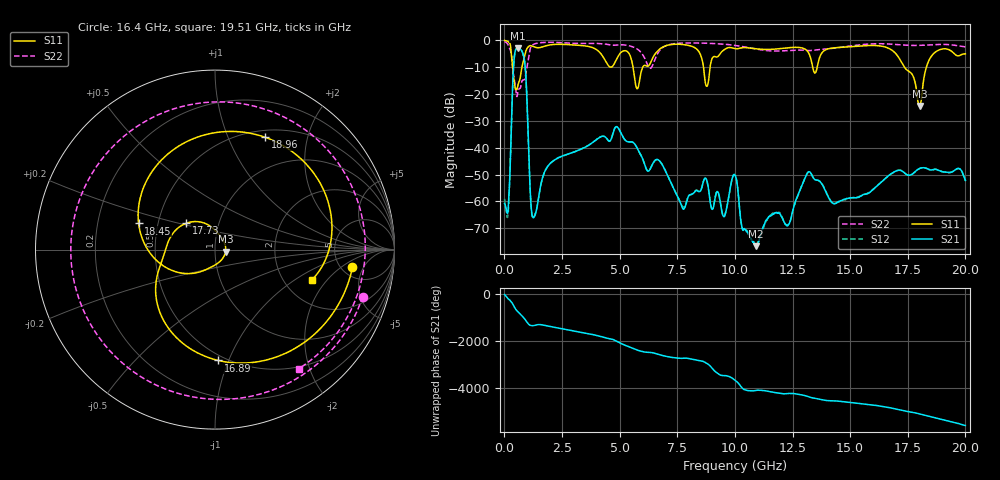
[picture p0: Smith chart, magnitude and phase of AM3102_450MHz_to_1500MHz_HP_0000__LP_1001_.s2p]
!Agilent Technologies,E8364B,MY43040894,A.07.50.67
!Agilent E8364B: A.07.50.67
!Date: Thursday, January 11, 2018 05:16:58
!Correction: S11(Full 2 Port(1,2))
!S21(Full 2 Port(1,2))
!S12(Full 2 Port(1,2))
!S22(Full 2 Port(1,2))
!S2P File: Measurements: S11, S21, S12, S22:
# Hz S  dB  R 50
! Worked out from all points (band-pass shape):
!   1601 points, 10 MHz to 20 GHz, reference 50 ohm
!   highest |S21| = -2.93 dB at 584.7 MHz (marker M1); lowest = -76.7 dB at 10.93 GHz (marker M2)
!   |S21| within 3 dB of the highest: 434.5 MHz to 835.3 MHz (400.8 MHz wide, 63.1 % of centre)
!   lowest |S11| = -24.5 dB at 18.01 GHz (marker M3), VSWR 1.13, Z = 56.2 - j1.29 ohm
!   |S11| at or under -10 dB: 355.9 MHz to 762.5 MHz (406.5 MHz wide, 72.7 % of centre); 5.581 GHz to 6.002 GHz (421.3 MHz wide, 7.28 % of centre); 17.35 GHz to 18.31 GHz (953 MHz wide, 5.34 % of centre)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
!   |S22| runs from -21.0 to -0.5 dB; largest |S21 - S12| = 0.0015
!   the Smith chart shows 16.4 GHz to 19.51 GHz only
!   S11 on the Smith chart (normalised r, x): 16.4 GHz: 6.27, -3.05; 16.89 GHz: 0.46, -0.92; 17.73 GHz: 0.70, +0.21; 18.45 GHz: 0.39, +0.14; 18.96 GHz: 0.58, +1.38; 19.51 GHz: 2.85, -1.40
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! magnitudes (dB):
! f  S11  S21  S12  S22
! 10 MHz  0.0  -60.8  -59.1  -0.5
! 172.4 MHz  -0.6  -61.6  -63.6  -1.9
! 409.8 MHz  -14.3  -8.4  -8.4  -13.6
! 584.7 MHz  -16.8  -2.9  -2.9  -19.1
! 884.6 MHz  -5.7  -8.3  -8.3  -14.5
! 1.259 GHz  -2.3  -66.1  -66.2  -1.5
! 3.346 GHz  -1.9  -40.5  -40.5  -1.2
! 5.757 GHz  -18.0  -40.1  -40.1  -3.2
! 6.682 GHz  -3.7  -44.6  -44.6  -4.4
! 7.756 GHz  -1.6  -62.8  -62.2  -1.0
! 10.01 GHz  -3.1  -50.2  -50.1  -1.9
! 10.93 GHz  -3.2  -76.7  -75.7  -3.3
! 13.34 GHz  -8.6  -50.3  -50.3  -3.8
! 16.4 GHz  -2.2  -52.4  -52.4  -1.3
! 16.68 GHz  -3.0  -50.4  -50.4  -1.4
! 16.89 GHz  -4.2  -49.1  -49.2  -1.5
! 17.73 GHz  -13.3  -49.6  -49.7  -1.9
! 18.01 GHz  -24.5  -47.7  -47.7  -1.9
! 18.45 GHz  -6.9  -48.2  -48.2  -1.7
! 18.96 GHz  -3.3  -48.9  -48.9  -1.5
! 19.51 GHz  -4.9  -48.6  -48.5  -1.8
! 20 GHz  -5.0  -52.2  -52.2  -2.4
